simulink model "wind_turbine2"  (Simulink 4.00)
settings: Solver=ode15s  StartTime=0.0  StopTime=600  RelTol=1e-4
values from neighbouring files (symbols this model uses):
  Awind = interp1(PointA(:,1),PointA(:,2), wmean)    [init.m]
  Bwind = interp1(PointB(:,1),PointB(:,2), wmean)    [init.m]
  Effy = 1.0    (= 1)    [init.m]
  g1 = DampLs    (= 15176)    [init.m]
  g2 = DampHs    (= 4.5112)    [init.m]
  gdash = GamLS    (= 265380)    [init.m]
  I1 = IneLs    (= 1029000)    [init.m]
  I2 = IneHs    (= 42.82)    [init.m]
  k1 = StfLs/(1+StfLs/StfHs/RatGB/RatGB)    (= 100437872.964)    [init.m]
  k2 = StfHs    (= 4850000)    [init.m]
  Kp = 29500    [init.m]
  Kv = 3200    [init.m]
  kw = 0.05    [init.m]
  N = RatGB    (= 58)    [init.m]
  OmLdic = RatGB*wref    (= 157.91718)    [init.m]
  OmlsIC = wref    (= 2.72271)    [init.m]
  RatedP = 1.0e6    (= 1000000)    [init.m]
  tau1 = beta/sqrt2    [init.m]
  tau2 = sqrta*beta/sqrt2    [init.m]
  tau3 = beta/sqrta    [init.m]
  TqlsIC = 219501.0    (= 219501)    [init.m]
  wmean = 5;init    [perf.m]    (also in tfs.m = 22; init; benchmark.m = 22; init)
  wref = 2.72271    [init.m]
libraries: simulink3 x1

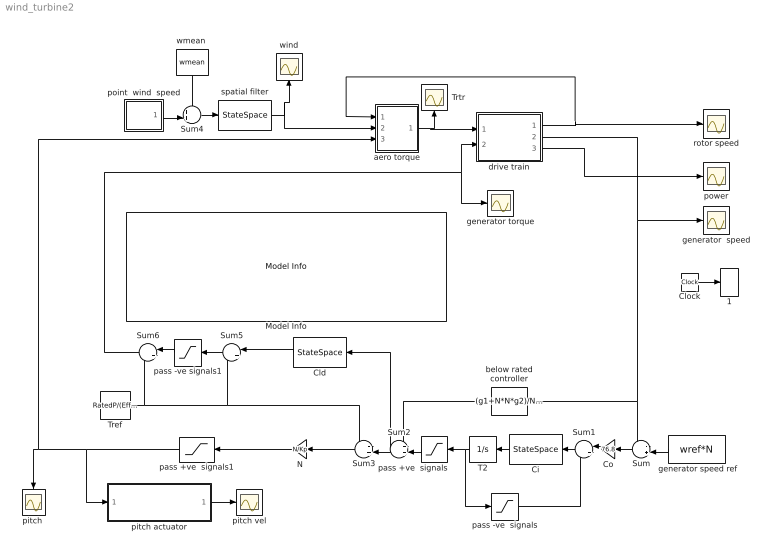
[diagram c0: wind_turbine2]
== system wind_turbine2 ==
  " generator speed ref" : Constant  Orientation=left  Value=wref*N
  1 : ToWorkspace  VariableName=t  SampleTime=-1  SaveFormat=Array
  Ci : StateSpace  Orientation=left  A=[-4 -3.5; 4 0]  B=[-31.25 ; 0]  C=[2.5 0.125]  D=0  X0=0  AbsoluteTolerance=auto  Realization=auto
  Cld : StateSpace  Orientation=left  A=-20  B=4  C=5  D=0  X0=0  AbsoluteTolerance=auto  Realization=auto
  Clock : Clock
  Co : Gain  Orientation=left  Gain=76.8  Multiplication=Element-wise(K.*u)  SaturateOnIntegerOverflow=on
  Model Info : simulink3/Signals & Systems/Model Info  InitialBlockCM=none  BlockCM=none  Frame=on  DisplayStringWithTags=|  HorizontalTextAlignment=Center  LeftAlignmentValue=0.5  SourceBlockDiagram=wind_turbine2  TagMaxNumber=20
      | WIND TURBINE BENCHMARK 
      | FOR HYBRID SYSTEM ANALYSIS & DESIGN
      | (c) D.J.Leith 2002
      | This software may be copied and freely distributed provided no changes 
      | are made (in particular this notice is not removed) and it is not used for 
      | commercial purposes without written permission.
  N : Gain  Orientation=left  Gain=N/Kp  Multiplication=Element-wise(K.*u)  SaturateOnIntegerOverflow=on
  Sum : Sum  Orientation=left  Inputs=-+|  SaturateOnIntegerOverflow=on
  Sum1 : Sum  Orientation=left  Inputs=|++  SaturateOnIntegerOverflow=on
  Sum2 : Sum  Orientation=left  Inputs=++|  SaturateOnIntegerOverflow=on
  Sum3 : Sum  Orientation=left  Inputs=-+|  SaturateOnIntegerOverflow=on
  Sum4 : Sum  Inputs=++|  SaturateOnIntegerOverflow=on
  Sum5 : Sum  Orientation=left  Inputs=|+-  SaturateOnIntegerOverflow=on
  Sum6 : Sum  Orientation=left  Inputs=|++  SaturateOnIntegerOverflow=on
  T2 : Integrator  Orientation=left  ExternalReset=none  InitialConditionSource=internal  InitialCondition=0  LimitOutput=off  UpperSaturationLimit=15e3  LowerSaturationLimit=0  ShowSaturationPort=off  ShowStatePort=off  AbsoluteTolerance=auto
  Tref : Constant  Value=RatedP/(Effy*wref*N)
  Trtr : Scope
  aero torque : Subsystem
  below rated controller : Fcn  Orientation=left  Expr=(g1+N*N*g2)/N*(u/N)
  drive train : Subsystem
  generator  speed : Scope
  generator torque : Scope
  pass +ve  signals : Saturate  Orientation=left  UpperLimit=1.0e9  LowerLimit=0  LinearizeAsGain=on
  pass +ve  signals1 : Saturate  Orientation=left  UpperLimit=1e9  LowerLimit=0  LinearizeAsGain=on
  pass -ve  signals : Saturate  UpperLimit=0  LowerLimit=-1.0e9  LinearizeAsGain=on
  pass -ve signals1 : Saturate  Orientation=left  UpperLimit=0  LowerLimit=-1.0e9  LinearizeAsGain=on
  "pitch " : Scope
  pitch actuator : Subsystem
  pitch vel : Scope
  point  wind  speed : Subsystem
  power : Scope
  rotor speed : Scope
  spatial filter : StateSpace  A="[0  1; -1/(tau2*tau3)   -(tau2+tau3)/(tau2*tau3)]"  B=[tau1/(tau2*tau3); (tau2*tau3-tau1*(tau2+tau3))/(tau2*tau3).^2]  C=[1 0]  D=0  X0=[wmean; -wmean*tau1/(tau2*tau3)]  AbsoluteTolerance=auto  Realization=auto
  wind : Scope
  "wmean " : Constant  Orientation=down  Value=wmean
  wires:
  " generator speed ref"/1 -> Sum/2
  Sum1/1 -> Ci/1
  pass -ve  signals/1 -> Sum1/2
  pass +ve  signals/1 -> Sum2/2
  Sum2/1 -> Sum3/2, Cld/1
  Ci/1 -> T2/1
  T2/1 -> pass +ve  signals/1, pass -ve  signals/1
  drive train/1(OmgLs) -> aero torque/1(OmgLs), rotor speed/1
  spatial filter/1 -> wind/1, aero torque/2(wind)
  aero torque/1(Trtr) -> Trtr/1, drive train/1(Trtr)
  N/1 -> pass +ve  signals1/1
  Sum/1 -> Co/1
  Co/1 -> Sum1/1
  Sum3/1 -> N/1
  below rated controller/1 -> Sum2/1
  Tref/1 -> Sum3/1, Sum5/2, Sum6/2
  Sum5/1 -> pass -ve signals1/1
  Sum6/1 -> drive train/2(TqLD), generator torque/1
  pass -ve signals1/1 -> Sum6/1
  Cld/1 -> Sum5/1
  Sum4/1 -> spatial filter/1
  "wmean "/1 -> Sum4/1
  pass +ve  signals1/1 -> aero torque/3(pitch), "pitch "/1, pitch actuator/1(pitch demand)
  pitch actuator/1(pitch vel) -> pitch vel/1
  Clock/1 -> 1/1
  drive train/3(power) -> power/1
  drive train/2(OmgLD) -> Sum/1, below rated controller/1, generator  speed/1
  point  wind  speed/1(point) -> Sum4/2

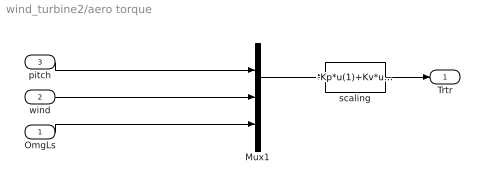
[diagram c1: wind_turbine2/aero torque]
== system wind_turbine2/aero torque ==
  OmgLs : Inport  Port=1  LatchInput=off
  wind : Inport  Port=2  LatchInput=off
  pitch : Inport  Port=3  LatchInput=off
  Mux1 : Mux  Inputs=3
  scaling : Fcn  Expr=-Kp*u(1)+Kv*u(2)*u(2)
  Trtr : Outport  Port=1
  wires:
  scaling/1 -> Trtr/1
  Mux1/1 -> scaling/1
  pitch/1 -> Mux1/1
  wind/1 -> Mux1/2
  OmgLs/1 -> Mux1/3

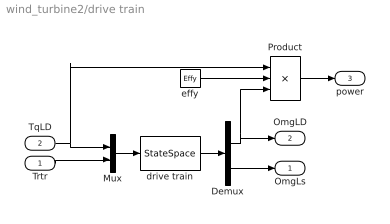
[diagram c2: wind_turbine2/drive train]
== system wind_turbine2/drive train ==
  Trtr : Inport  Port=1  LatchInput=off
  TqLD : Inport  Port=2  LatchInput=off
  Demux : Demux  Outputs=2  BusSelectionMode=off
  Mux : Mux  Inputs=2
  Product : Product  Inputs=3  Multiplication=Element-wise(.*)  SaturateOnIntegerOverflow=on
  drive train : StateSpace  A=[-g2/I2 1/N/I2 0; -k1/N 0 k1; (gdash/N-gdash*k1/N/N/N/k2)/I1 -1/I1 -(g1+gdash-gdash*k1/N/N/k2)/I1]  B=[-1/I2 0;0 0; 0 1/I1]  C=[1 0 0; 0 0 1]  D=[0 0;0 0]  X0=[OmLdic TqlsIC OmlsIC]  AbsoluteTolerance=auto  Realization=auto
  effy : Constant  Value=Effy
  OmgLs : Outport  Port=1
  OmgLD : Outport  Port=2
  power : Outport  Port=3
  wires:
  Mux/1 -> drive train/1
  Trtr/1 -> Mux/2
  drive train/1 -> Demux/1
  Demux/2 -> OmgLs/1
  TqLD/1 -> Mux/1, Product/1
  Demux/1 -> OmgLD/1, Product/3
  effy/1 -> Product/2
  Product/1 -> power/1

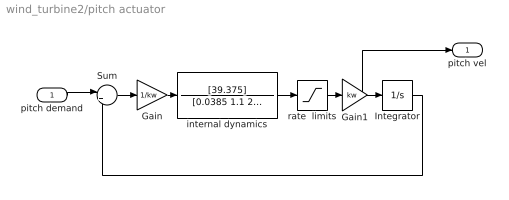
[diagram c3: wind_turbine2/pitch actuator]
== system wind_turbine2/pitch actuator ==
  pitch demand : Inport  Port=1  LatchInput=off
  Gain : Gain  Gain=1/kw  Multiplication=Element-wise(K.*u)  SaturateOnIntegerOverflow=on
  Gain1 : Gain  Gain=kw  Multiplication=Element-wise(K.*u)  SaturateOnIntegerOverflow=on
  Integrator : Integrator  ExternalReset=none  InitialConditionSource=internal  InitialCondition=0  LimitOutput=off  UpperSaturationLimit=inf  LowerSaturationLimit=-inf  ShowSaturationPort=off  ShowStatePort=off  AbsoluteTolerance=auto
  Sum : Sum  Inputs=|+-  SaturateOnIntegerOverflow=on
  internal dynamics : TransferFcn  Numerator=[39.375]  Denominator=[0.0385 1.1 20.475]  AbsoluteTolerance=auto  Realization=auto
  rate  limits : Saturate  UpperLimit=1e9  LowerLimit=-1e9  LinearizeAsGain=on
  pitch vel : Outport  Port=1
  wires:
  pitch demand/1 -> Sum/1
  Sum/1 -> Gain/1
  Gain/1 -> internal dynamics/1
  internal dynamics/1 -> rate  limits/1
  rate  limits/1 -> Gain1/1
  Integrator/1 -> Sum/2
  Gain1/1 -> Integrator/1, pitch vel/1

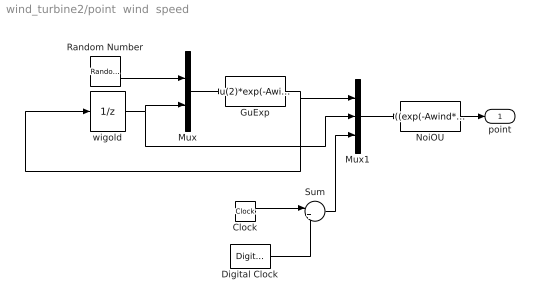
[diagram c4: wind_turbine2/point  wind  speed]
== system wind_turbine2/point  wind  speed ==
  Clock : Clock
  Digital Clock : DigitalClock  SampleTime=0.02
  GuExp : Fcn  Expr=u(2)*exp(-Awind*0.02)+Bwind*u(1)*sqrt((1.-exp(-Awind*0.02))*(1.+exp(-Awind*0.02))/(2*Awind))
  Mux : Mux  Inputs=2
  Mux1 : Mux  Inputs=3
  NoiOU : Fcn  Expr=((exp(-Awind*u(3))-exp(-Awind*0.02))*(1.+exp(-Awind*(0.02-u(3))))*u(2)+ (exp(-Awind*(0.02-u(3)))-exp(-Awind*0.02))*(1.0+exp(-Awind*u(3)))*u(1))/(1.-exp(-Awind*0.02))/(1.0+exp(-Awind*0.02))
  Random Number : RandomNumber  Mean=0  Variance=1  Seed=55  SampleTime=0.02
  Sum : Sum  Inputs=|+-  SaturateOnIntegerOverflow=on
  wigold : UnitDelay  X0=0  SampleTime=0.02
  point : Outport  Port=1
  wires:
  Random Number/1 -> Mux/1
  Mux/1 -> GuExp/1
  Clock/1 -> Sum/1
  Digital Clock/1 -> Sum/2
  NoiOU/1 -> point/1
  Mux1/1 -> NoiOU/1
  Sum/1 -> Mux1/3
  wigold/1 -> Mux/2, Mux1/2
  GuExp/1 -> Mux1/1, wigold/1
